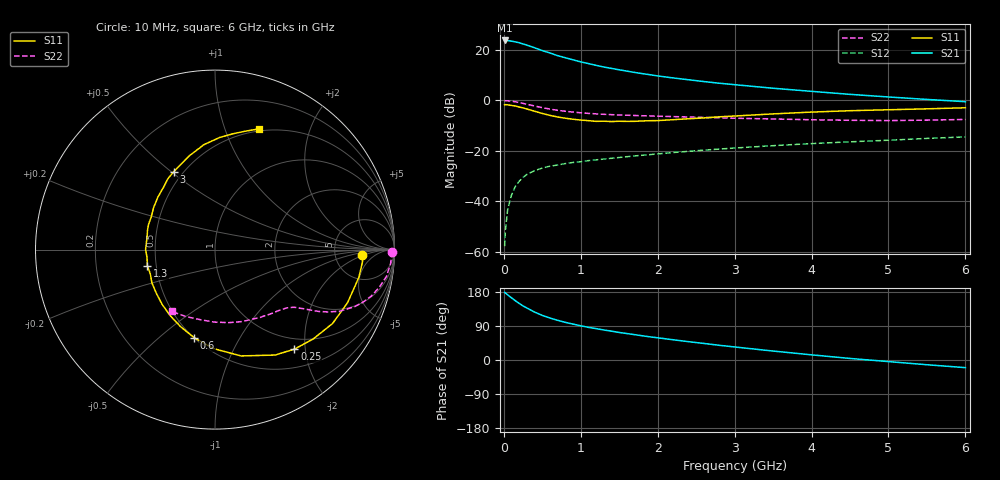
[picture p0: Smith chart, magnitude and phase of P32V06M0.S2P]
! SIEMENS Small Signal Semiconductors
! BFP181
! Si NPN RF Bipolar Junction Transistor in SOT143
! VCE = 2 V  IC = 6 mA
! Common Emitter S-Parameters:  March  1996
# GHz  S  MA  R  50
!  f  S11  S21  S12  S22
! GHz  MAG  ANG  MAG  ANG  MAG  ANG  MAG  ANG
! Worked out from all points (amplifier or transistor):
!   36 points, 10 MHz to 6 GHz, reference 50 ohm
!   highest |S21| = 23.7 dB at 10 MHz (marker M1)
!   |S21| within 3 dB of that: start of sweep to 409.5 MHz
!   unconditionally stable (mu >= 1): 1.436 GHz to end of sweep
!   at 250 MHz: K = 0.26, MSG = 26.4 dB, |S12| = -30.5 dB
!   at 1.4 GHz: K = 0.99, MSG = 17.8 dB, |S12| = -22.9 dB
!   at 6 GHz: K = 1.03, MAG = 6.0 dB, |S12| = -14.5 dB
!   S11 on the Smith chart (normalised r, x): 10 MHz: 9.69, -1.85; 250 MHz: 0.80, -1.79; 600 MHz: 0.50, -0.66; 1.3 GHz: 0.45, -0.10; 3 GHz: 0.45, +0.51; 6 GHz: 0.48, +1.31
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0.01  0.819 -2.2  15.39 178.4  0.0013 85.8  0.9873 -0.7
0.02  0.8249 -4.6  15.33 177.1  0.0026 87.2  0.9852 -1.8
0.05  0.8164 -10.9  15.29 171.9  0.007 84.1  0.9814 -4.6
0.1  0.7957 -21.8  14.9 164.0  0.0134 77.3  0.9671 -8.9
0.15  0.7736 -32.2  14.41 156.3  0.0199 73.1  0.9393 -12.9
0.2  0.7398 -42.3  13.87 149.2  0.0251 68.7  0.9093 -16.5
0.25  0.7095 -51.4  13.12 142.7  0.0299 64.0  0.8733 -19.7
0.3  0.6763 -60.3  12.42 137.2  0.0342 60.4  0.8393 -22.3
0.4  0.61 -76.2  11.03 126.4  0.0407 54.8  0.7748 -26.3
0.5  0.5515 -90.9  9.697 117.7  0.0458 50.9  0.7187 -28.9
0.6  0.5048 -103.2  8.674 110.7  0.05 47.6  0.673 -30.8
0.7  0.4699 -114.2  7.689 104.7  0.0526 46.0  0.6358 -32.1
0.8  0.4438 -124.6  6.991 99.3  0.0562 44.6  0.6097 -33.1
1.1  0.3974 -152.2  5.363 86.1  0.0643 42.5  0.5537 -35.6
1.3  0.3878 -166.4  4.586 79.2  0.069 41.6  0.531 -37.4
1.7  0.3852 168.9  3.582 66.9  0.0795 41.2  0.5031 -41.4
2.2  0.4153 145.3  2.787 53.4  0.0928 39.5  0.4783 -47.6
3  0.4908 118.1  2.049 34.4  0.1141 36.1  0.4439 -59.9
3.5  0.5408 105.5  1.742 23.6  0.1271 33.4  0.429 -69.1
4.5  0.6253 87.6  1.318 4.1  0.1513 26.7  0.4039 -90.7
5.5  0.6812 75.6  1.046 -12.5  0.1768 20.5  0.4068 -113.5
6  0.715 70.1  0.944 -20.2  0.1894 16.6  0.4201 -125.1
